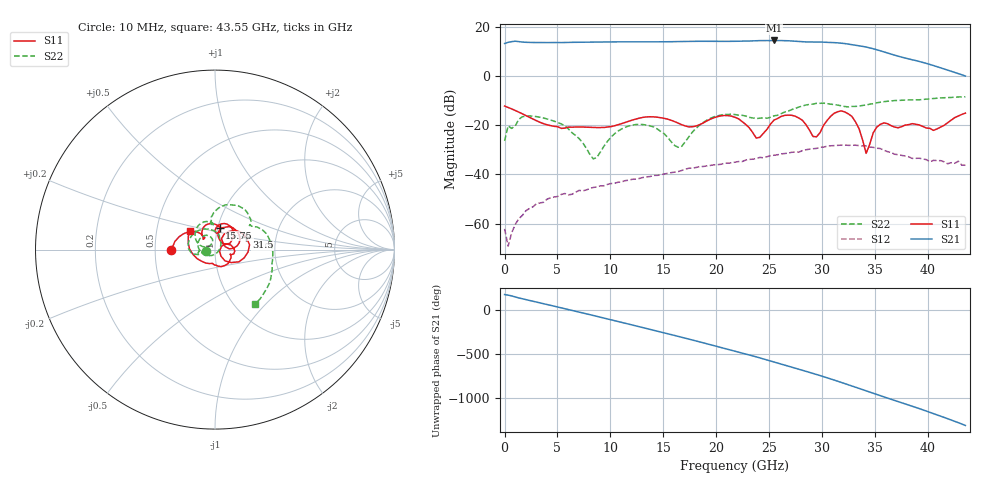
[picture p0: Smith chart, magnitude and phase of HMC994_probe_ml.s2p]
! Hittite Microwave Corporation
! 2 Elizabeth Drive
! Chelmsford, MA 01824
! http://www.hittite.com
! Tel: 978-250-3343
! Fax: 978-250-3373
! Device:  HMC994
! Description: GaAs pHEMT MMIC 0.5 Watt Power Amplifier
! Frequency:  DC - 32.00 GHz
! Package:  DIE
! Ports:  2 RF, 3 DC
!  Pad  1 = RF Input  = Port 1
!  Pad  2 = Vgg2
!  Pad  3 = ACG1
!  Pad  4 = ACG2
!  Pad  5 = RF Output, Vdd = POrt 2
!  Pad  6 = ACG3
!  Pad  7 = ACG4
!  Pad  8 = Vgg1
! Voltages:  Vdd = +10.00 Volts, Idd = +249.96 mA
!  Vg1 =  -0.48 Volts, Ig1 =  -0.01 mA
!  Vg2 =  +3.50 Volts, Ig2 =  +0.05 mA
! Data:  The device was measured using G-S-G Probes on a microstrip
!  alumina launch.  The launch is 0.25 inches long. 3 mil Ribbon bonds
!  of approximately 15 mils in length connected the launcher to the die.
!  NO DE_EMBEDDING WAS DONE.
!  Data was collected using an calibrated network analyzer.
!  The reference plane is the microstrip launcher.
! Misc:  Validation Unit  2, +25 C
! Date Measured:  ~2011-05-01
! Date:  2011-08-30 MJV
! Note:
!  Hittite supplies this data as a sample of measured data at the microstrip
!  launch.  Your particular data for this product may vary.
!  Data was taken at 25 degrees C.
!  Hittite reserves the right to change this data at anytime.
# GHZ S DB R 50.0
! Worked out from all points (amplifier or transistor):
!   131 points, 10 MHz to 43.55 GHz, reference 50 ohm
!   highest |S21| = 14.4 dB at 25.47 GHz (marker M1)
!   |S21| within 3 dB of that: start of sweep to 34.51 GHz
!   unconditionally stable (mu >= 1): start of sweep to end of sweep
!   at 7.044 GHz: K = 21.79, MAG = 13.7 dB, |S12| = -46.5 dB
!   at 21.78 GHz: K = 5.39, MAG = 14.2 dB, |S12| = -35.0 dB
!   at 43.55 GHz: K = 27.44, MAG = 0.7 dB, |S12| = -36.3 dB
!   S11 on the Smith chart (normalised r, x): 10 MHz: 0.61, -0.00; 15.75 GHz: 1.02, +0.25; 31.5 GHz: 1.41, +0.20; 43.55 GHz: 0.74, +0.16
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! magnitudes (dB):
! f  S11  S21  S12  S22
! 10 MHz  -12.3  13.1  -62.1  -26.4
! 344.9 MHz  -12.8  13.6  -69.1  -20.3
! 1.015 GHz  -14.1  14.1  -60.4  -20.3
! 2.355 GHz  -16.8  13.6  -53.9  -16.3
! 7.379 GHz  -20.8  13.6  -46.7  -27.1
! 8.384 GHz  -20.9  13.7  -45.3  -33.7
! 11.4 GHz  -18.9  13.8  -42.5  -20.9
! 14.75 GHz  -17.0  13.8  -40.1  -22.5
! 15.75 GHz  -18.0  13.9  -39.3  -26.8
! 16.76 GHz  -19.9  13.9  -38.4  -28.6
! 21.78 GHz  -16.8  14.0  -35.0  -15.7
! 23.79 GHz  -25.3  14.3  -33.5  -17.3
! 25.47 GHz  -18.0  14.4  -32.2  -16.2
! 27.48 GHz  -16.4  14.0  -31.0  -13.2
! 29.15 GHz  -24.6  13.7  -29.6  -11.5
! 31.5 GHz  -14.6  13.4  -28.3  -11.9
! 32.84 GHz  -16.5  12.6  -28.2  -12.4
! 34.17 GHz  -31.5  11.7  -28.5  -11.9
! 35.18 GHz  -20.8  10.6  -29.4  -10.9
! 36.52 GHz  -20.2  8.8  -31.0  -10.2
! 40.54 GHz  -22.1  4.2  -34.3  -9.2
! 43.55 GHz  -15.1  -0.1  -36.3  -8.5
